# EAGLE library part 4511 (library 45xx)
BCD to 7-segment LATCH/DECODER/DRIVER
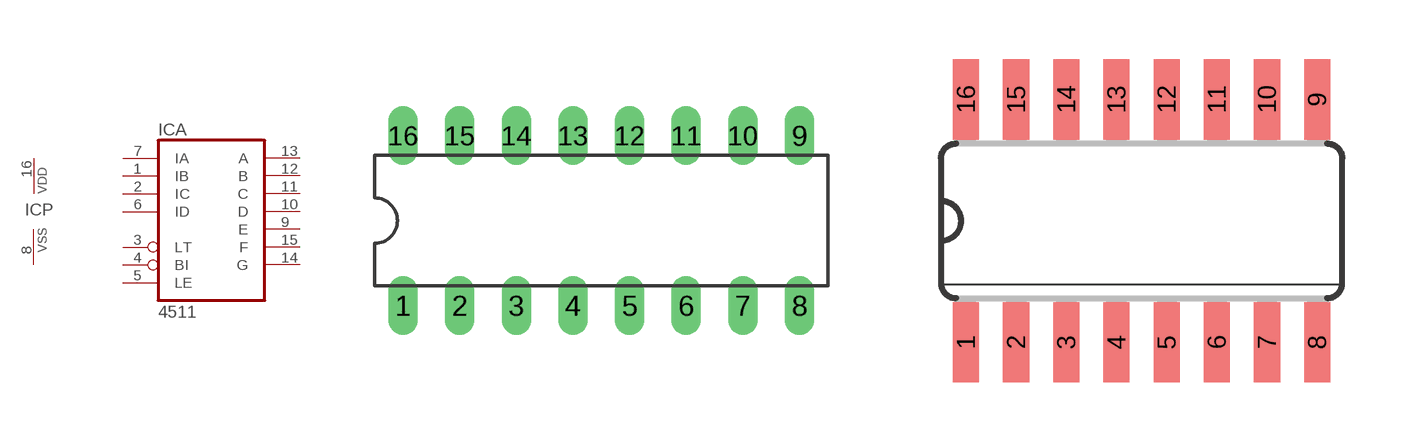
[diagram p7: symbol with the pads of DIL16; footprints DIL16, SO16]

Designator prefix IC; gates A=4511 P=PWRN

## 4511N  [DIL16]
1  A:IB  in
2  A:IC  in
3  A:LT  in
4  A:BI  in
5  A:LE  in
6  A:ID  in
7  A:IA  in
8  P:VSS  pwr
9  A:E  out
10  A:D  out
11  A:C  out
12  A:B  out
13  A:A  out
14  A:G  out
15  A:F  out
16  P:VDD  pwr

## 4511D  [SO16]
Pads as for DIL16

## Footprint DIL16 (pad centres in mm)
Dual In Line Package
drill 0.813 long: 1 -8.89,-3.81; 2 -6.35,-3.81; 3 -3.81,-3.81; 4 -1.27,-3.81; 5 1.27,-3.81; 6 3.81,-3.81; 7 6.35,-3.81; 8 8.89,-3.81; 9 8.89,3.81; 10 6.35,3.81; 11 3.81,3.81; 12 1.27,3.81; 13 -1.27,3.81; 14 -3.81,3.81; 15 -6.35,3.81; 16 -8.89,3.81

## Footprint SO16 (pad centres in mm)
Small Outline package 150 mil
smd 0.66 x 2.032: 1 -4.445,-3.073; 2 -3.175,-3.073; 3 -1.905,-3.073; 4 -0.635,-3.073; 5 0.635,-3.073; 6 1.905,-3.073; 7 3.175,-3.073; 8 4.445,-3.073; 9 4.445,3.073; 10 3.175,3.073; 11 1.905,3.073; 12 0.635,3.073; 13 -0.635,3.073; 14 -1.905,3.073; 15 -3.175,3.073; 16 -4.445,3.073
